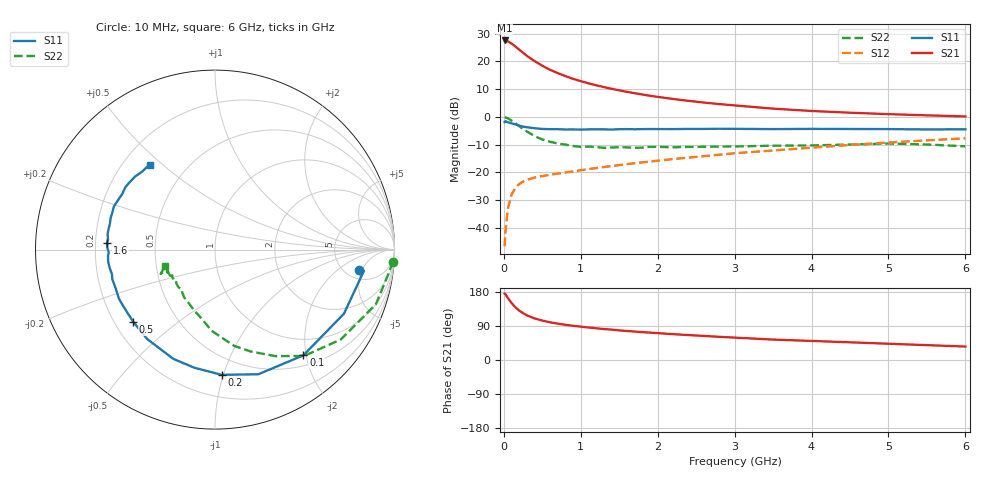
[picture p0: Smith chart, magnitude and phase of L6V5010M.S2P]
!  INFINEON TECHNOLOGIES Small Signal Semiconductors
! BFR380L3 , Si-NPN RF-Transistor in TSLP-3-1
!  Vce=0.5 V,  Ic=10 mA
! Common Emitter S-Parameters:  07. March 2005
#  GHz  S  MA  R  50
! f  S11  S21  S12  S22
! GHz  Mag  Ang  Mag  Ang  Mag  Ang  Mag  Ang
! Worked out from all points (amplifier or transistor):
!   36 points, 10 MHz to 6 GHz, reference 50 ohm
!   highest |S21| = 27.5 dB at 10 MHz (marker M1)
!   |S21| within 3 dB of that: start of sweep to 186.5 MHz
!   unconditionally stable (mu >= 1): 1.895 GHz to 5.88 GHz
!   at 250 MHz: K = 0.29, MSG = 23.2 dB, |S12| = -23.3 dB
!   at 1.4 GHz: K = 0.92, MSG = 13.9 dB, |S12| = -17.7 dB
!   at 6 GHz: K = 1.00, MSG = 3.9 dB, |S12| = -7.7 dB
!   S11 on the Smith chart (normalised r, x): 10 MHz: 6.65, -4.27; 100 MHz: 0.68, -1.95; 200 MHz: 0.36, -0.99; 500 MHz: 0.28, -0.35; 1.6 GHz: 0.25, +0.03; 6 GHz: 0.31, +0.45
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0.01  0.8083 -7.9  23.82 175.1  0.0047 82.9  0.9933 -3.9
0.02  0.8382 -8.1  23.71 173.9  0.0083 86.9  0.9763 -7.8
0.05  0.8024 -26.4  23.02 164.3  0.0215 78.2  0.9469 -18.7
0.1  0.7678 -50.1  20.97 150.6  0.0398 66.5  0.8618 -35.5
0.15  0.7353 -70.8  18.61 139.1  0.0527 57.3  0.7727 -50.1
0.2  0.6987 -87.0  16.26 130.3  0.0618 52.4  0.6819 -60.5
0.25  0.6679 -100.0  14.29 123.6  0.0685 47.7  0.6001 -70.9
0.3  0.6515 -110.9  12.57 117.9  0.0735 45.2  0.5465 -78.8
0.4  0.6253 -127.2  10.1 109.7  0.0808 41.8  0.4524 -92.4
0.5  0.6077 -138.5  8.361 104.1  0.0861 41.4  0.3917 -101.0
0.6  0.6006 -147.1  7.06 99.5  0.0907 41.7  0.3572 -109.1
0.8  0.5937 -158.9  5.432 92.9  0.0996 43.2  0.317 -122.8
0.9  0.5956 -163.9  4.848 90.3  0.1041 44.6  0.2991 -127.8
1.1  0.5962 -170.3  4.028 85.7  0.1149 46.8  0.2924 -134.0
1.3  0.5971 -176.6  3.449 81.7  0.1252 48.3  0.2774 -141.5
1.6  0.6026 176.3  2.827 76.5  0.1412 50.8  0.2826 -147.9
2.2  0.603 166.2  2.104 68.2  0.1743 54.1  0.2839 -151.4
2.8  0.612 157.4  1.704 61.2  0.2084 56.2  0.292 -156.2
3.5  0.6028 148.8  1.409 53.9  0.2485 55.9  0.3028 -156.1
4.5  0.6058 141.8  1.191 46.7  0.3125 55.8  0.3183 -156.2
5.5  0.5948 133.0  1.067 39.2  0.3781 52.8  0.3185 -157.7
6  0.5981 127.6  1.021 35.5  0.4116 50.9  0.295 -162.0
